PROGRAM MAIN

VAR CONSTANT 
	cInitMA : ST_MA_MultiArray_InitPars := (eTypeCode := eMA_TypeCode_LREAL, nDims := 2, aDimSizes := [cChannels, cBufferLength]);
END_VAR

VAR
	// Signal generation
	fbFunctionGenerator			: FB_FunctionGenerator;		// signal generator
	fSetFrequency				: LREAL := 50;				// Hz
	fSetAmplitude				: LREAL := 5;				// peak amplitude of sin signal
	eFunction					: E_FunctionType :=  E_FunctionType.Sine;
	
	// signal buffer
	aBuffer                     : ARRAY[1..cOversamples] OF LREAL;	
	p 							: UDINT;
	aEl3632						: ARRAY[1..cOversamples] OF INT;
	nSelectInput				: INT := 1;
	
	// MA Buffer
	fbSource                   : FB_CMA_Source := (stInitPars := cInitMA,
											       nOwnID     := eID_Source,
											       aDestIDs   := [eID_RMS]);
											   
	fbSink   				   : FB_CMA_Sink := (nOwnID := eID_Sink);											   
											   
	fbErrHist			       : FB_HRErrHist; // error monitoring		
	
	bRMSBufferSent			   : BOOL;         // Boolean indicating a transfer to FB_CMA_RMS
	bNewRMSvalue  			   : BOOL;	       // Boolean indicating a new RMS Value ready in PlcTask
	aRmsResult				   : ARRAY [1..cChannels] OF LREAL;
   
END_VAR

// signal input
CASE nSelectInput OF	
	1:  // From internal signal generator
			fbFunctionGenerator(	bEnable	:= TRUE,
									fFrequency 	:= fSetFrequency,
									fAmplitude 	:= fSetAmplitude,
									fOffset 	:= ,
									nDutyCycle	:= ,
									eFunction 	:= eFunction,
									aSignal		:= aBuffer ); 
	2:  // Measurement unit: g
		FOR p := 1 TO cOversamples DO
			aBuffer[p] := INT_TO_LREAL(aEl3632[p]);				
		END_FOR
END_CASE

// call source
fbSource.Input2D(	pDataIn:= ADR(aBuffer), 
					nDataInSize:= SIZEOF(aBuffer), 
					eElementType:= eMA_TypeCode_LREAL, 
					nWorkDim0:= 0, 
					nWorkDim1:= 1, 
					pStartIndex:= 0, 
					nOptionPars:= 0, 
					bNewResult=> bRMSBufferSent, 
					bError=> , 
					hrErrorCode=> );
IF fbSource.bError THEN
	fbErrHist.AddError(bErr := TRUE, hrErrCode := fbSource.hrErrorCode, sErrSource := 'MAIN.fbSource.Input2D');
END_IF
				  
// call sink				  
fbSink.Output1D(	pDataOut	:= ADR(aRmsResult), 
					nDataOutSize:= SIZEOF(aRmsResult), 
					eElementType:= eMA_TypeCode_LREAL, 
					nWorkDim	:= 0, 
					nElements	:= 0, 
					pStartIndex	:= 0, 
					nOptionPars	:= 0, 
					bNewResult	=> bNewRMSvalue, 
					bError		=> , 
					hrErrorCode	=> );		
IF fbSink.bError THEN
	fbErrHist.AddError(bErr := TRUE, hrErrCode := fbSink.hrErrorCode, sErrSource := 'MAIN.fbSink.Output1D');
END_IF

END_PROGRAM
